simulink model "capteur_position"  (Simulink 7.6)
settings: Solver=ode15s  StartTime=0.0  StopTime=5  RelTol=1e-3
InitFcn:
  | clear all
  | clc
  | close all
StopFcn:
  | close all, clc
  | load position_recopie.mat
  | plotyy(x(1,:),x(2,:), x(1,:),x(3,:))
  | grid
  | title('position et sa recopie par potentiomètre linéaire')
  | xlabel('temps')
libraries: elec_lib x3, nesl_utility x3, fl_lib x2

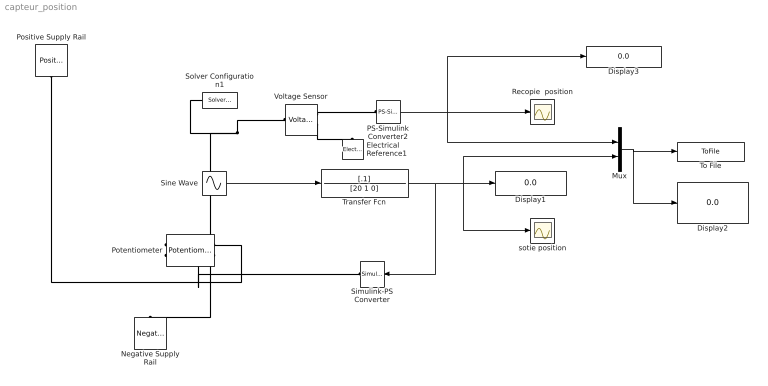
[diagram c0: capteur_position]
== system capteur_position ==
  Display1 : Display
  Display2 : Display
  Display3 : Display
  Electrical Reference1 : fl_lib/Electrical/Electrical Elements/Electrical Reference  DialogController=NetworkEngine.DynNeDlgSource  SystemSampleTime=-1  i_Log=off  LocalVarNames=|i  LocalVarDescs=|i  LocalVarLogging=[]
  Mux : Mux  Inputs=2
  Negative Supply Rail : elec_lib/Sources/Negative Supply Rail  DialogController=NetworkEngine.DynNeDlgSource  SystemSampleTime=-1  v0=-12 V  current_Log=off  voltage_Log=off  power_Log=off  LocalVarNames=|current|voltage|power  LocalVarDescs=|Current (A)|Voltage (V)|Power (W)  LocalVarLogging=[0 0 0]
  PS-Simulink Converter2 : nesl_utility/PS-Simulink Converter  DialogController=NetworkEngine.DynNeUtilDlgSource  SystemSampleTime=-1  PhysicalDomain=network_engine_domain  LeftPortType=input  RightPortType=output  SubClassName=ps_output  Unit=1  AffineConversion=off
  Positive Supply Rail : elec_lib/Sources/Positive Supply Rail  DialogController=NetworkEngine.DynNeDlgSource  SystemSampleTime=-1  v0=12 V  current_Log=off  voltage_Log=off  power_Log=off  LocalVarNames=|current|voltage|power  LocalVarDescs=|Current (A)|Voltage (V)|Power (W)  LocalVarLogging=[0 0 0]
  Potentiometer : elec_lib/Passive Devices/Potentiometer  DialogController=NetworkEngine.DynNeDlgSource  SystemSampleTime=-1  R0=10e3 Ohm  Rw=1e-22 Ohm  Rcenter=200 Ohm  xmin=0  xmax=1  Taper=1  Gradient=1  LocalVarLogging=[]
  Recopie  position : Scope
  Simulink-PS Converter : nesl_utility/Simulink-PS Converter  DialogController=NetworkEngine.DynNeUtilDlgSource  SystemSampleTime=-1  PhysicalDomain=network_engine_domain  LeftPortType=input  RightPortType=output  SubClassName=ps_input  Unit=1  AffineConversion=off  InputFilterTimeConstant=.001  UdotUserProvided=0
  Sine Wave : Sin  Bias=1  SampleTime=0
  Solver Configuration1 : nesl_utility/Solver Configuration  DialogController=NetworkEngine.DynNeUtilDlgSource  SystemSampleTime=-1  PhysicalDomain=network_engine_domain  LeftPortType=input  RightPortType=generic  SubClassName=solver  Accelerate=off  Profile=off  ResidualTolerance=1e-9  MaxNonlinIter=12  MaxModeIter=2  DoFixedCost=off  UseLocalSampling=off  DoDC=off  LinearAlgebra=Sparse  LocalSolverSampleTime=.001  LocalSolverChoice=NE_BACKWARD_EULER_ADVANCER  UseLocalSolver=off
  To File : ToFile  Filename=position_recopie  MatrixName=x
  Transfer Fcn : TransferFcn  Numerator=[.1]  Denominator=[20 1 0]
  Voltage Sensor : fl_lib/Electrical/Electrical Sensors/Voltage Sensor  DialogController=NetworkEngine.DynNeDlgSource  SystemSampleTime=-1  i1_Log=off  v1_Log=off  LocalVarNames=|i1|v1  LocalVarDescs=|i1|v1  LocalVarLogging=[0 0]
  sotie position : Scope
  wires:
  Sine Wave/1 -> Transfer Fcn/1
  Transfer Fcn/1 -> Simulink-PS Converter/1, Display1/1, sotie position/1, Mux/2
  PS-Simulink Converter2/1 -> Recopie  position/1, Mux/1, Display3/1
  Mux/1 -> To File/1, Display2/1
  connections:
  Potentiometer/LConn2 -- Voltage Sensor/LConn1 -- Solver Configuration1/RConn1
  Voltage Sensor/RConn1 -- PS-Simulink Converter2/LConn1
  Voltage Sensor/RConn2 -- Electrical Reference1/LConn1
  Potentiometer/LConn1 -- Negative Supply Rail/LConn1
  Positive Supply Rail/RConn1 -- Potentiometer/RConn1
  Potentiometer/RConn2 -- Simulink-PS Converter/RConn1
